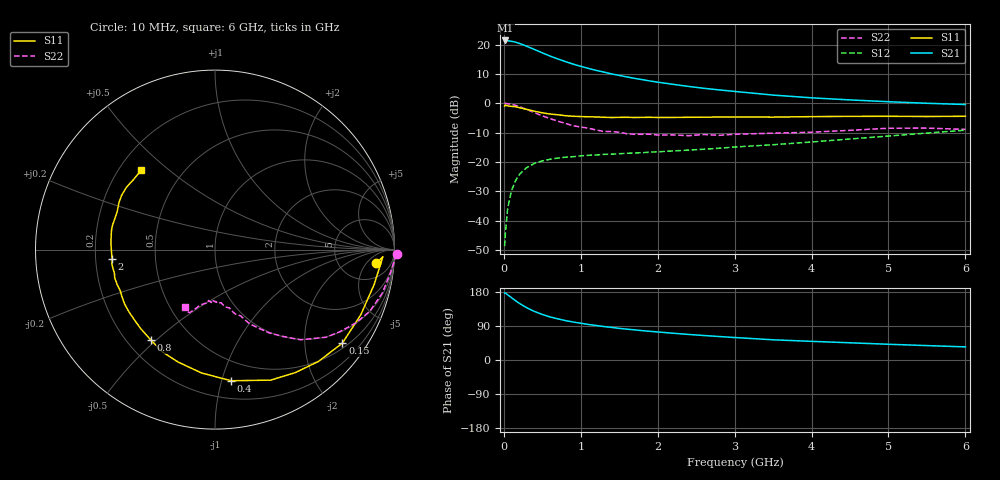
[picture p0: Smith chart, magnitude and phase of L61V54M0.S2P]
!  INFINEON TECHNOLOGIES Small Signal Semiconductors
! BFR380L3 , Si-NPN RF-Transistor in TSLP-3-1
!  Vce=1.5 V,  Ic=4 mA
! Common Emitter S-Parameters:  07. March 2005
#  GHz  S  MA  R  50
! f  S11  S21  S12  S22
! GHz  Mag  Ang  Mag  Ang  Mag  Ang  Mag  Ang
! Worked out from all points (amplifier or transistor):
!   36 points, 10 MHz to 6 GHz, reference 50 ohm
!   highest |S21| = 21.5 dB at 20 MHz (marker M1)
!   |S21| within 3 dB of that: start of sweep to 391.2 MHz
!   unconditionally stable (mu >= 1): 2.52 GHz to 4.783 GHz
!   at 250 MHz: K = 0.14, MSG = 21.4 dB, |S12| = -22.9 dB
!   at 1.4 GHz: K = 0.71, MSG = 13.7 dB, |S12| = -17.3 dB
!   at 6 GHz: K = 0.95, MSG = 4.4 dB, |S12| = -9.1 dB
!   S11 on the Smith chart (normalised r, x): 10 MHz: 11, -9; 150 MHz: 0.63, -2.93; 400 MHz: 0.34, -1.07; 800 MHz: 0.30, -0.48; 2 GHz: 0.27, -0.04; 6 GHz: 0.29, +0.40
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0.01  0.9001 -4.9  11.81 176.7  0.0037 88.9  1.013 -1.5
0.02  0.9365 -2.4  11.82 177.1  0.0062 90.3  1.003 -3.2
0.05  0.9077 -12.4  11.71 172.0  0.0163 83.9  0.9867 -7.4
0.1  0.8897 -24.1  11.42 164.4  0.0329 77.8  0.9632 -14.6
0.15  0.8803 -36.3  11.09 156.8  0.0477 70.8  0.9287 -21.7
0.2  0.8489 -47.2  10.55 149.7  0.0609 66.3  0.8857 -27.4
0.25  0.8187 -56.8  9.983 143.6  0.0717 61.0  0.8337 -33.2
0.3  0.7907 -66.9  9.377 137.6  0.0809 56.7  0.7891 -38.2
0.4  0.7362 -83.0  8.274 127.8  0.0955 50.0  0.6927 -46.5
0.5  0.6912 -96.3  7.27 120.3  0.1048 46.0  0.614 -52.0
0.6  0.6595 -108.1  6.412 113.7  0.1117 42.2  0.5517 -57.1
0.8  0.6174 -125.4  5.163 104.0  0.1211 38.5  0.4559 -65.0
0.9  0.6046 -133.0  4.674 100.2  0.1238 37.5  0.4168 -67.5
1.1  0.5921 -143.7  3.946 93.7  0.1308 36.8  0.378 -72.3
1.5  0.5789 -160.5  2.999 83.5  0.139 37.8  0.3228 -80.1
2  0.576 -174.8  2.3 74.0  0.1499 41.0  0.2892 -89.0
2.2  0.5768 -178.8  2.114 70.6  0.155 42.7  0.2914 -89.2
2.8  0.5865 169.5  1.698 61.9  0.1724 47.9  0.2861 -97.3
3.5  0.5842 159.0  1.387 53.3  0.1978 52.1  0.311 -102.6
4.5  0.6017 149.9  1.147 45.4  0.2476 57.6  0.348 -108.5
5.5  0.5986 139.4  1.006 38.0  0.3126 58.9  0.3797 -114.5
6  0.6039 133.1  0.957 34.6  0.3494 58.1  0.3607 -118.1
